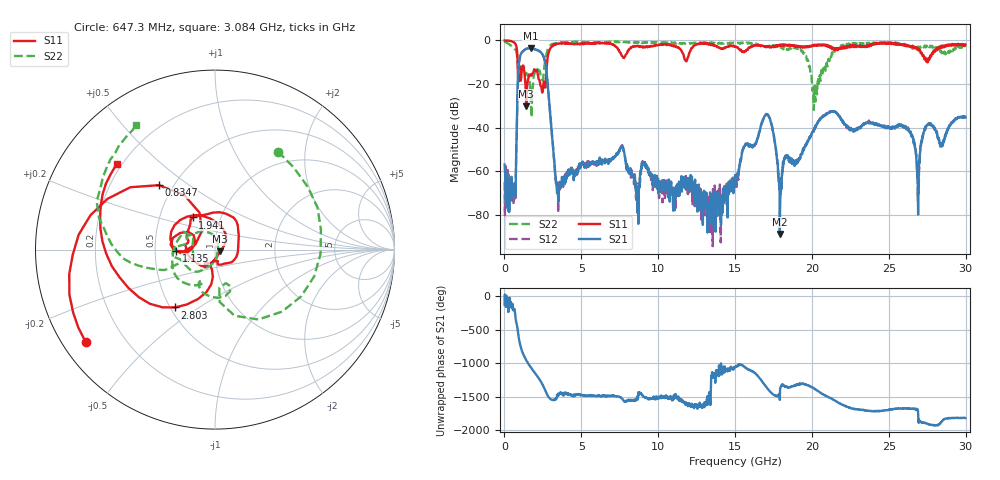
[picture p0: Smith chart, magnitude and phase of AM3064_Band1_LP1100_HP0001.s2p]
# Hz S DB R 50.0
!freq dBS11 angS11 dBS21 angS21 dBS12 angS12 dBS22 angS22
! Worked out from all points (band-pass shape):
!   1600 points, 10 MHz to 29.98 GHz, reference 50 ohm
!   highest |S21| = -3.63 dB at 1.716 GHz (marker M1); lowest = -88.6 dB at 17.91 GHz (marker M2)
!   |S21| within 3 dB of the highest: 1.046 GHz to 2.495 GHz (1.449 GHz wide, 81.9 % of centre)
!   lowest |S11| = -30.2 dB at 1.416 GHz (marker M3), VSWR 1.06, Z = 53 - j1.08 ohm
!   |S11| at or under -10 dB: 857.6 MHz to 2.775 GHz (1.917 GHz wide, 106 % of centre); 27.52475 GHz to 27.52999 GHz (5.24 MHz wide, 0.019 % of centre)
!   |S22| runs from -35.2 to -0.4 dB; largest |S21 - S12| = 0.0089
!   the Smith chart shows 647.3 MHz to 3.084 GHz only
!   S11 on the Smith chart (normalised r, x): 647.3 MHz: 0.07, -0.32; 834.7 MHz: 0.42, +0.39; 1.135 GHz: 0.64, -0.01; 1.941 GHz: 0.73, +0.28; 2.803 GHz: 0.53, -0.40; 3.084 GHz: 0.18, +0.36
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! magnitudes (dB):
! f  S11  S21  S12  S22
! 10 MHz  0.0  -56.9  -64.8  -0.4
! 647.3 MHz  -1.1  -65.4  -68.0  -3.8
! 834.7 MHz  -6.4  -27.6  -27.5  -8.3
! 1.135 GHz  -13.3  -5.5  -5.4  -13.1
! 1.416 GHz  -30.2  -3.9  -3.8  -15.8
! 1.716 GHz  -15.8  -3.6  -3.7  -25.9
! 1.941 GHz  -13.2  -4.0  -4.0  -15.4
! 2.803 GHz  -8.1  -19.4  -19.3  -4.3
! 3.084 GHz  -2.8  -43.0  -42.7  -1.7
! 3.496 GHz  -1.5  -69.1  -78.9  -1.1
! 5.015 GHz  -1.4  -56.1  -56.4  -0.6
! 7.62 GHz  -6.9  -48.2  -48.4  -0.7
! 8.651 GHz  -2.6  -79.0  -75.8  -0.9
! 10 GHz  -2.1  -70.1  -62.8  -1.0
! 15 GHz  -2.8  -61.6  -64.3  -1.3
! 17.05 GHz  -2.8  -33.8  -33.7  -3.0
! 17.91 GHz  -2.0  -88.6  -69.2  -3.0
! 19.99 GHz  -2.8  -42.7  -42.6  -18.2
! 25 GHz  -1.1  -39.5  -39.7  -1.2
! 26.89 GHz  -3.8  -68.5  -73.4  -3.3
! 27.53 GHz  -10.0  -38.5  -38.5  -3.1
! 29.98 GHz  -1.9  -35.2  -35.1  -3.0
